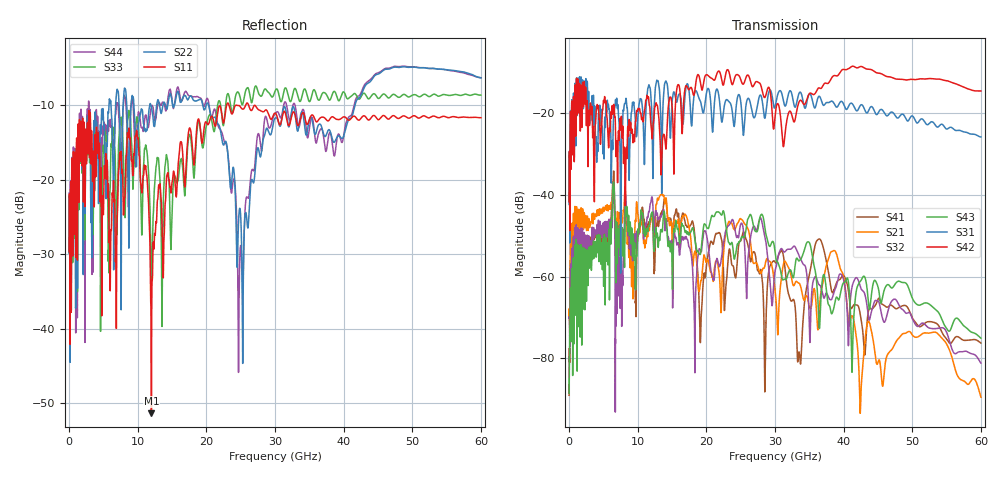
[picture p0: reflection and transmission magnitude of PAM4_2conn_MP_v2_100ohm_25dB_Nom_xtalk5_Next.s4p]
! Info: Touchstone file created by Circ.  Input file=FAB50GbE_2conn_Midplane_Examax_Topo2_v2_100ohm_25dB_Nom.circ
# Hz S RI R 50
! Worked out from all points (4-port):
!   6000 points, 10 MHz to 60 GHz, reference 50 ohm
!   strongest paths, dB at 10 MHz, 15.01 GHz, 30.01 GHz, 45.01 GHz, 60 GHz:
!     S42: -41.7, -18.2, -20.8, -10.2, -14.6
!     S31: -42.4, -17.3, -18.5, -20.0, -25.8
!     S43: -88.5, -56.0, -53.9, -62.5, -75.1
!     S32: -70.1, -54.9, -58.6, -66.0, -81.2
!     S21: -69.8, -49.6, -63.3, -81.0, -89.5
!     S41: -89.1, -48.3, -56.5, -65.6, -76.3
!   lowest |S11| = -51.3 dB at 12 GHz (marker M1), VSWR 1.01, Z = 50.1 + j0.236 ohm
!   |S11| at or under -10 dB: start of sweep to 22.97 GHz; 23.29 GHz to 25.74 GHz (2.447 GHz wide, 9.98 % of centre); 26.15 GHz to end of sweep
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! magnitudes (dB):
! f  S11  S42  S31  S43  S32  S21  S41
! 10 MHz  -29.7  -41.7  -42.4  -88.5  -70.1  -69.8  -89.1
! 12 GHz  -51.3  -23.7  -17.8  -44.5  -40.9  -45.7  -45.2
! 18.32 GHz  -17.0  -14.6  -14.9  -50.8  -80.9  -53.9  -49.9
! 24.87 GHz  -10.2  -11.1  -15.8  -51.5  -48.3  -45.9  -51.3
! 33.54 GHz  -12.5  -17.2  -15.0  -56.1  -55.0  -61.7  -78.6
! 36.39 GHz  -12.0  -13.8  -15.9  -70.5  -61.9  -70.3  -50.8
! 60 GHz  -11.7  -14.6  -25.8  -75.1  -81.2  -89.5  -76.3
